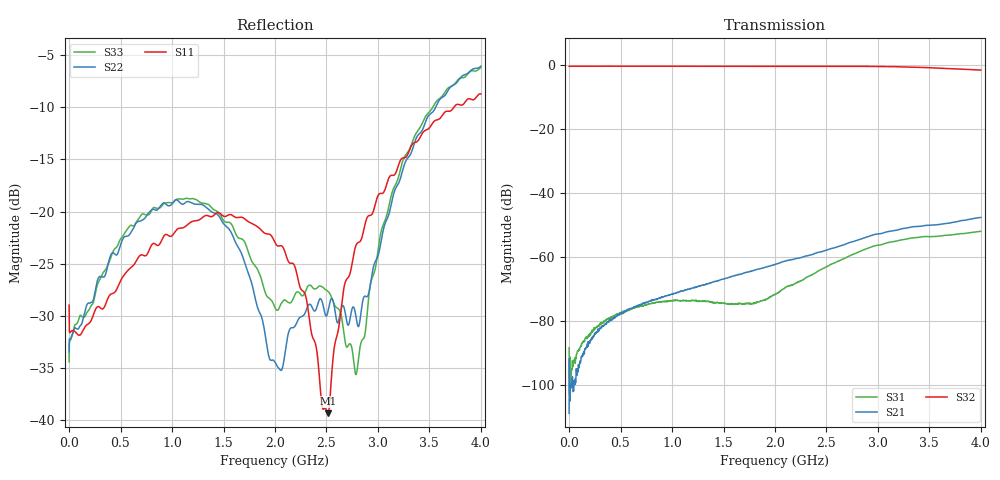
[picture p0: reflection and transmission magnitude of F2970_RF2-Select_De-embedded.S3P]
! Integrated Device Technology
! Corporate Headquarters
! 6024 Silver Creek Valley Road
! San Jose, CA 95138  USA
! Phone:  1-408-284-8200
! Toll Free:  1-800-223-1366
! Webpage:  http://www.idt.com/
! Timing and RF Division
! 515 Groton Road, Suite 102
! Westford, MA 01886-6024
! Device:  F2970
! Description: 75 Ohm SP2T RF Switch
! Frequency:  5.0 -  3000.00 MHz
! Package:  4x4 mm LQFN Plastic Package: 20 pin
! Ports:  3 RF, 2 DC
!  Pin  1  = GND
!  Pin  2  = GND
!  Pin  3  = RF1  = Port 1
!  Pin  4  = GND
!  Pin  5  = GND
!  Pin  6  = GND
!  Pin  7  = GND
!  Pin  8  = RFC  = Port 3
!  Pin  9  = GND
!  Pin 10  = GND
!  Pin 11  = GND
!  Pin 12  = GND
!  Pin 13  = RF2  = Port 2
!  Pin 14  = GND
!  Pin 15  = GND
!  Pin 16  = C2
!  Pin 17  = C1
!  Pin 18  = GND
!  Pin 19  = GND
!  Pin 20  = VCC
! State:  RF2 Selected
! Voltage:  Vcc = +3.0 Volts
!  C1 = +3.0 V,  C2 = 0.0 V
! Data:  The device was measured on a the F2970 evaluation board which has
!  individual transmission lines to the RF pins.  Data was collected
!  using a calibrated network analyzer.  The evaluation board was
!  de-embedded using a PORT EXTENSTION technique.
!  The reference plane is the edge of the package pin.
! Misc:
!  Action Tracker AT0363
! Date Measured:  2014-11-08
! Date:  2016-11-29  MJV
! Note:
!  Integrated Device Technology supplies this data as a sample of measured
!  data at the package pin for this product.  Your particular data for this
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# Hz S dB R 75
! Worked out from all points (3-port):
!   1601 points, 300 kHz to 4 GHz, reference 75 ohm
!   strongest paths, dB at 300 kHz, 1 GHz, 2 GHz, 3 GHz, 4 GHz:
!     S32: -0.3, -0.3, -0.3, -0.3, -1.4
!     S21: -108.8, -71.5, -62.3, -52.7, -47.5
!     S31: -88.3, -73.6, -71.6, -56.2, -51.9
!   lowest |S11| = -39.4 dB at 2.515 GHz (marker M1), VSWR 1.02, Z = 73.9 - j1.2 ohm
!   |S11| at or under -10 dB: start of sweep to 3.736 GHz
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300000  -28.99 159.5  -97.86 -0.4  -94.91 -113.3
        -108.81 -58.5  -33.48 34.2  -0.28 0.7
        -88.33 -117.0  -0.27 0.7  -34.43 26.5
5.60258e8  -25.78 -112.0  -76.74 105.7  -76.71 83.8
           -76.69 106.1  -22.37 -80.5  -0.25 -7.5
           -76.68 82.7  -0.25 -7.5  -21.76 -78.7
1.042722e9  -21.77 -88.2  -71.19 120.2  -73.47 92.3
            -71.15 120.0  -18.86 -95.9  -0.29 -13.3
            -73.45 91.5  -0.30 -13.3  -18.84 -90.7
1.567682e9  -20.29 -66.0  -66.10 138.1  -74.53 123.1
            -66.09 138.4  -21.88 -96.1  -0.30 -19.5
            -74.67 121.9  -0.30 -19.5  -21.11 -86.3
2.00015e9  -22.98 -51.4  -62.27 149.3  -71.57 177.4
           -62.27 149.4  -34.47 -30.8  -0.28 -25.0
           -71.62 177.6  -0.28 -25.0  -29.24 -30.1
2.292628e9  -27.94 -48.2  -59.69 154.4  -66.54 -163.5
            -59.68 154.4  -29.74 31.7  -0.29 -28.7
            -66.58 -163.4  -0.29 -28.7  -27.76 14.2
2.515111e9  -39.37 -131.0  -57.60 158.2  -62.72 -158.8
            -57.59 158.3  -29.57 12.6  -0.28 -31.5
            -62.76 -158.4  -0.28 -31.6  -27.67 16.9
2.790091e9  -23.17 -177.6  -54.77 159.6  -58.66 -160.4
            -54.77 159.7  -30.30 -35.2  -0.28 -35.4
            -58.65 -160.3  -0.28 -35.5  -35.61 -53.3
3.250056e9  -14.84 -169.6  -50.99 150.7  -54.45 -175.6
            -50.98 150.8  -15.69 -129.5  -0.42 -42.8
            -54.45 -175.6  -0.44 -42.8  -14.90 -136.8
4e9  -8.70 -139.0  -47.54 144.2  -51.86 179.0
     -47.53 144.3  -6.04 -140.4  -1.42 -51.4
     -51.87 179.2  -1.45 -51.3  -6.16 -137.8
